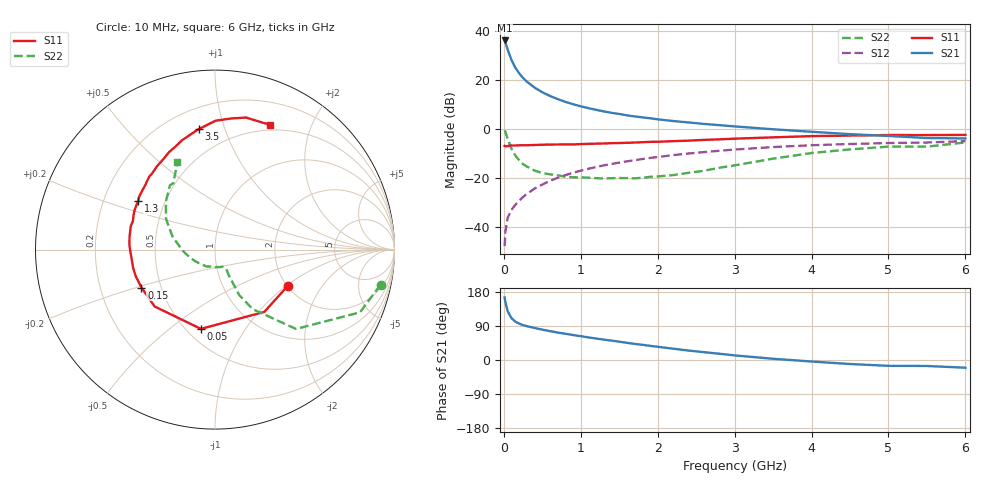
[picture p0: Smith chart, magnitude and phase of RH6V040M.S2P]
! SIEMENS Small Signal Semiconductors
! BFR106
! Si NPN RF Bipolar Junction Transistor in SOT23
! VCE = 6 V  IC = 40 mA
! Common Emitter S-Parameters:  August  1996
# GHz  S  MA  R  50
!  f  S11  S21  S12  S22
! GHz  MAG  ANG  MAG  ANG  MAG  ANG  MAG  ANG
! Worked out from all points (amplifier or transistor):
!   36 points, 10 MHz to 6 GHz, reference 50 ohm
!   highest |S21| = 36.3 dB at 10 MHz (marker M1)
!   |S21| within 3 dB of that: start of sweep to 42.58 MHz
!   unconditionally stable (mu >= 1): 279.1 MHz to 2.193 GHz
!   at 250 MHz: K = 0.98, MSG = 24.4 dB, |S12| = -27.8 dB
!   at 1.4 GHz: K = 1.06, MAG = 9.0 dB, |S12| = -14.3 dB
!   at 6 GHz: K = 0.98, MSG = 0.5 dB, |S12| = -4.9 dB
!   S11 on the Smith chart (normalised r, x): 10 MHz: 2.00, -1.03; 50 MHz: 0.59, -0.65; 150 MHz: 0.39, -0.21; 1.3 GHz: 0.35, +0.26; 3.5 GHz: 0.33, +0.82; 6 GHz: 0.44, +1.44
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0.01  0.4526 -26.8  65.33 165.2  0.004 82.9  0.9429 -12.0
0.02  0.4427 -51.6  60.15 153.3  0.0078 74.9  0.8801 -23.4
0.05  0.4487 -100.1  42.43 128.6  0.0153 61.5  0.632 -44.4
0.1  0.4621 -136.7  25.88 110.3  0.0223 59.2  0.3936 -57.6
0.15  0.4609 -152.7  18 101.1  0.0282 61.4  0.2862 -62.0
0.2  0.4658 -161.4  13.83 96.0  0.034 65.1  0.2295 -61.8
0.25  0.4674 -167.5  11.12 92.0  0.0408 66.4  0.1908 -61.9
0.3  0.4667 -172.2  9.326 89.2  0.0472 68.7  0.1708 -62.0
0.4  0.4724 -179.1  7.072 84.5  0.0604 70.3  0.1412 -60.9
0.5  0.4783 176.4  5.675 80.1  0.0731 70.9  0.1258 -59.9
0.6  0.4813 171.5  4.76 76.2  0.0871 70.7  0.1185 -61.0
0.7  0.4836 167.6  4.11 72.4  0.1005 70.1  0.1126 -63.3
0.9  0.4842 160.8  3.225 65.9  0.1276 68.4  0.1031 -66.7
1.1  0.4989 154.0  2.684 59.6  0.154 66.3  0.101 -75.4
1.3  0.5071 147.7  2.301 53.7  0.1808 63.8  0.0976 -83.2
1.7  0.5302 136.9  1.817 42.5  0.2308 58.6  0.098 -105.1
2.2  0.5659 124.8  1.464 29.9  0.2927 51.5  0.1141 -135.4
2.8  0.6158 110.7  1.205 16.5  0.3593 42.7  0.161 -170.4
3.5  0.6769 97.8  0.991 3.2  0.4286 32.4  0.2479 162.9
4.5  0.737 82.7  0.788 -10.6  0.4949 17.5  0.3839 135.4
5.5  0.7546 70.5  0.656 -15.8  0.5303 7.6  0.4368 122.1
6  0.7597 66.3  0.644 -20.4  0.5678 0.3  0.5326 113.1
